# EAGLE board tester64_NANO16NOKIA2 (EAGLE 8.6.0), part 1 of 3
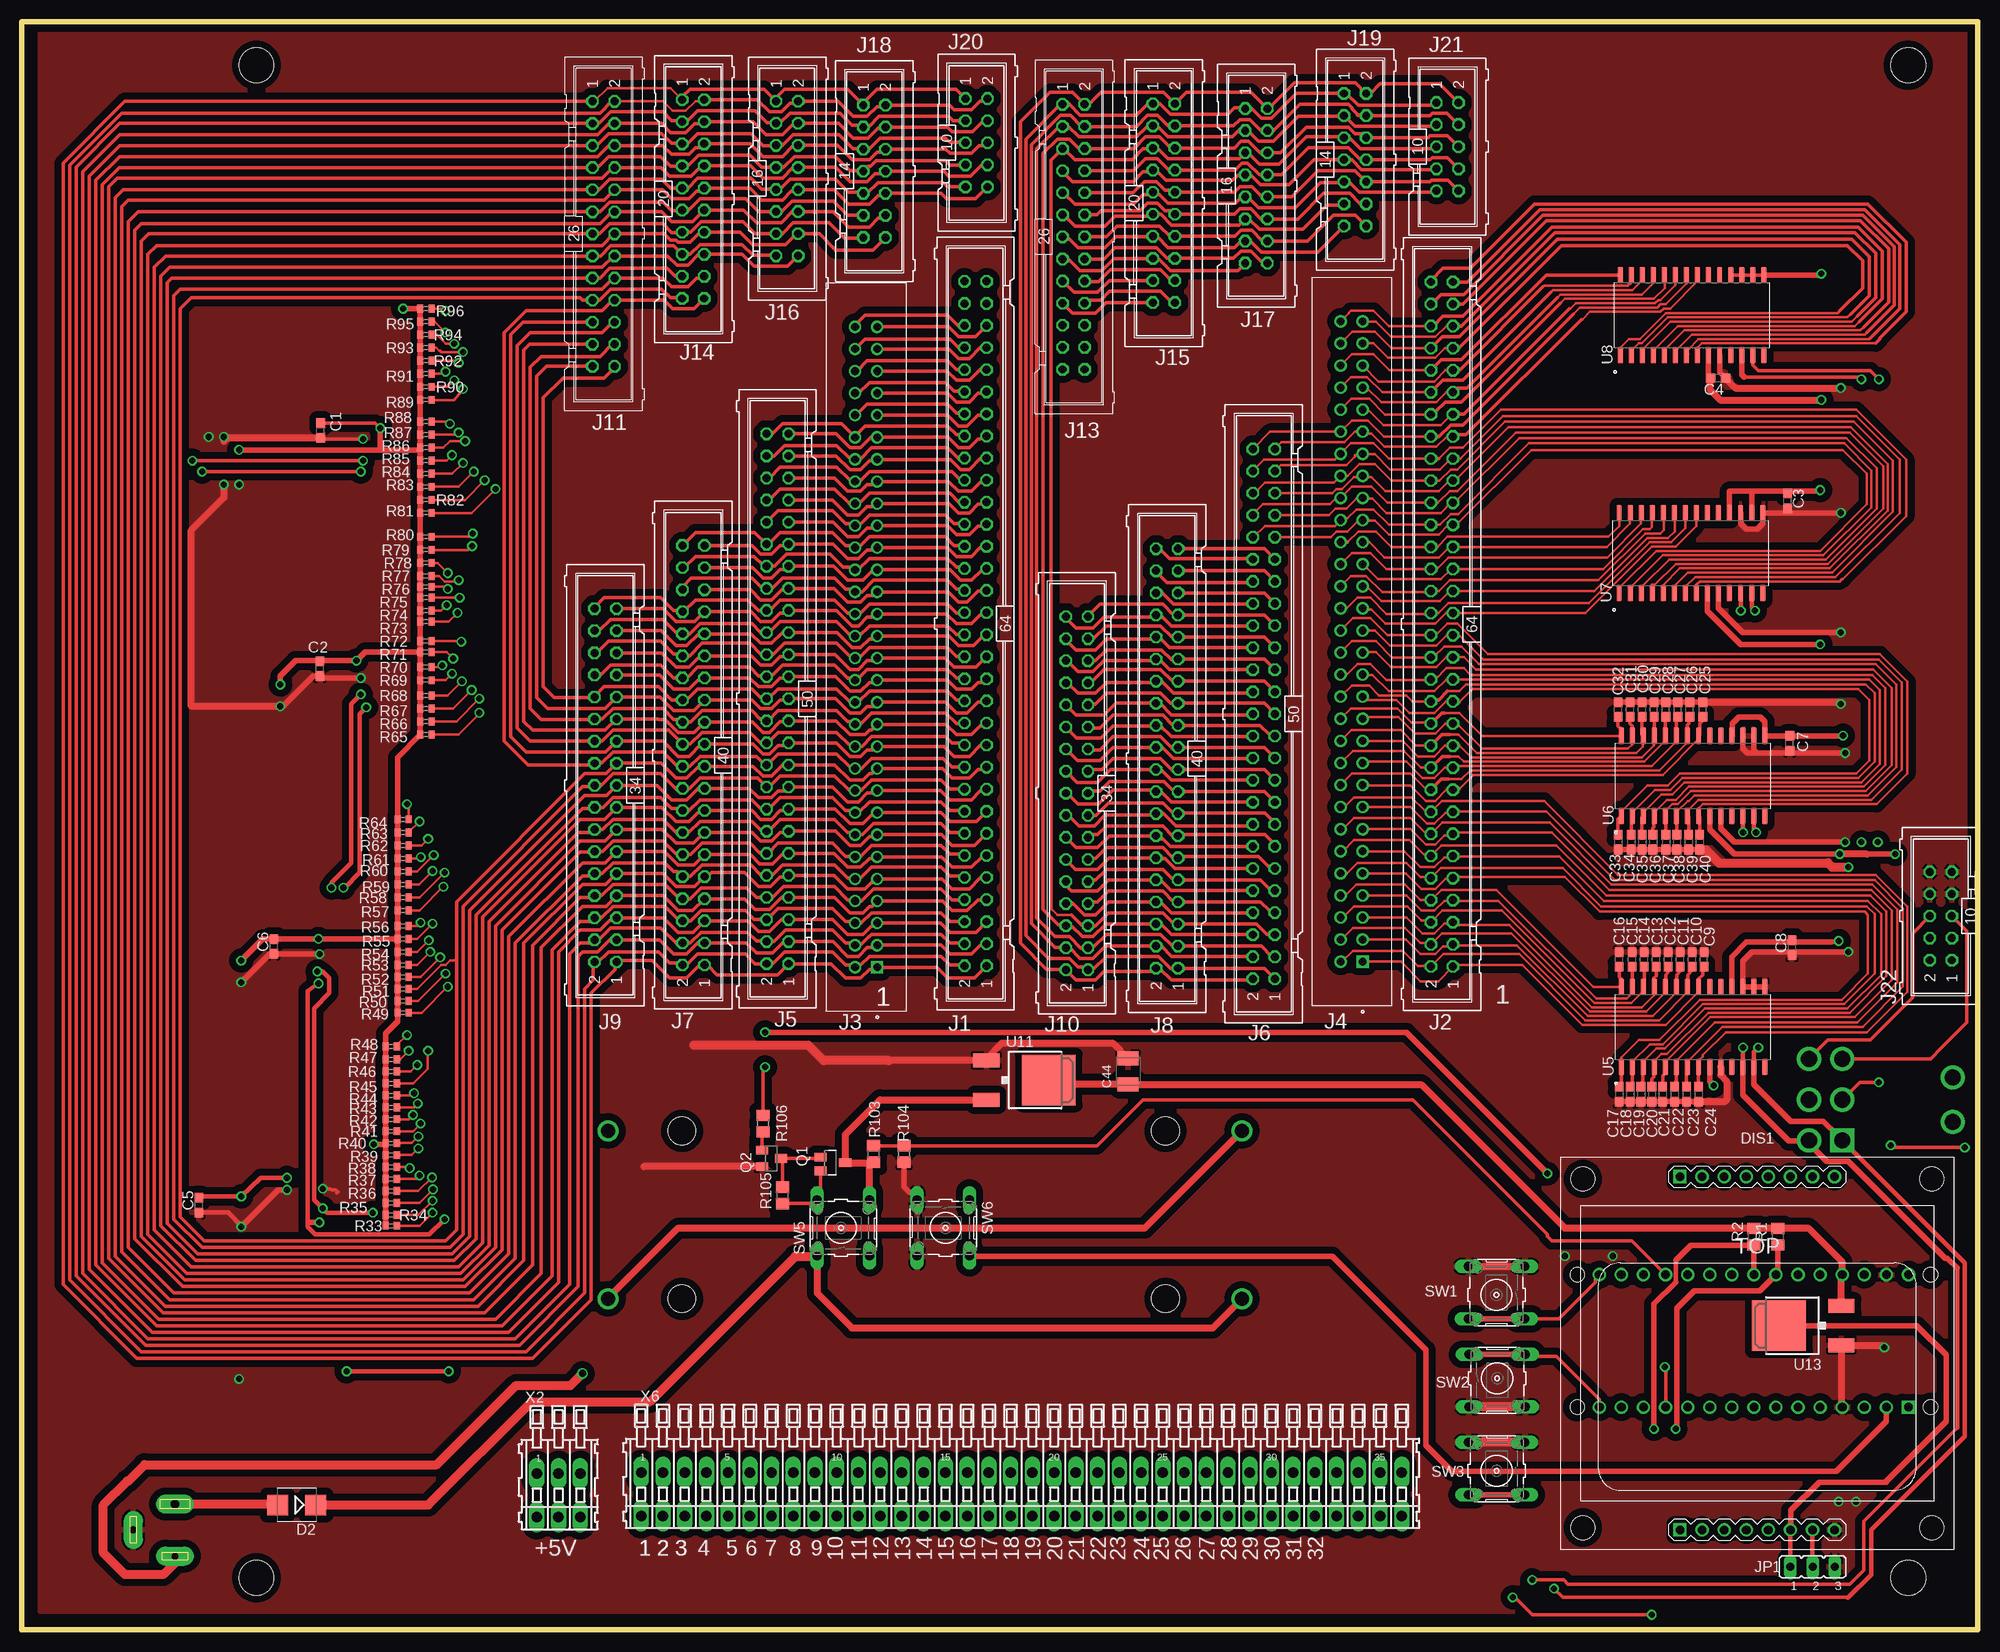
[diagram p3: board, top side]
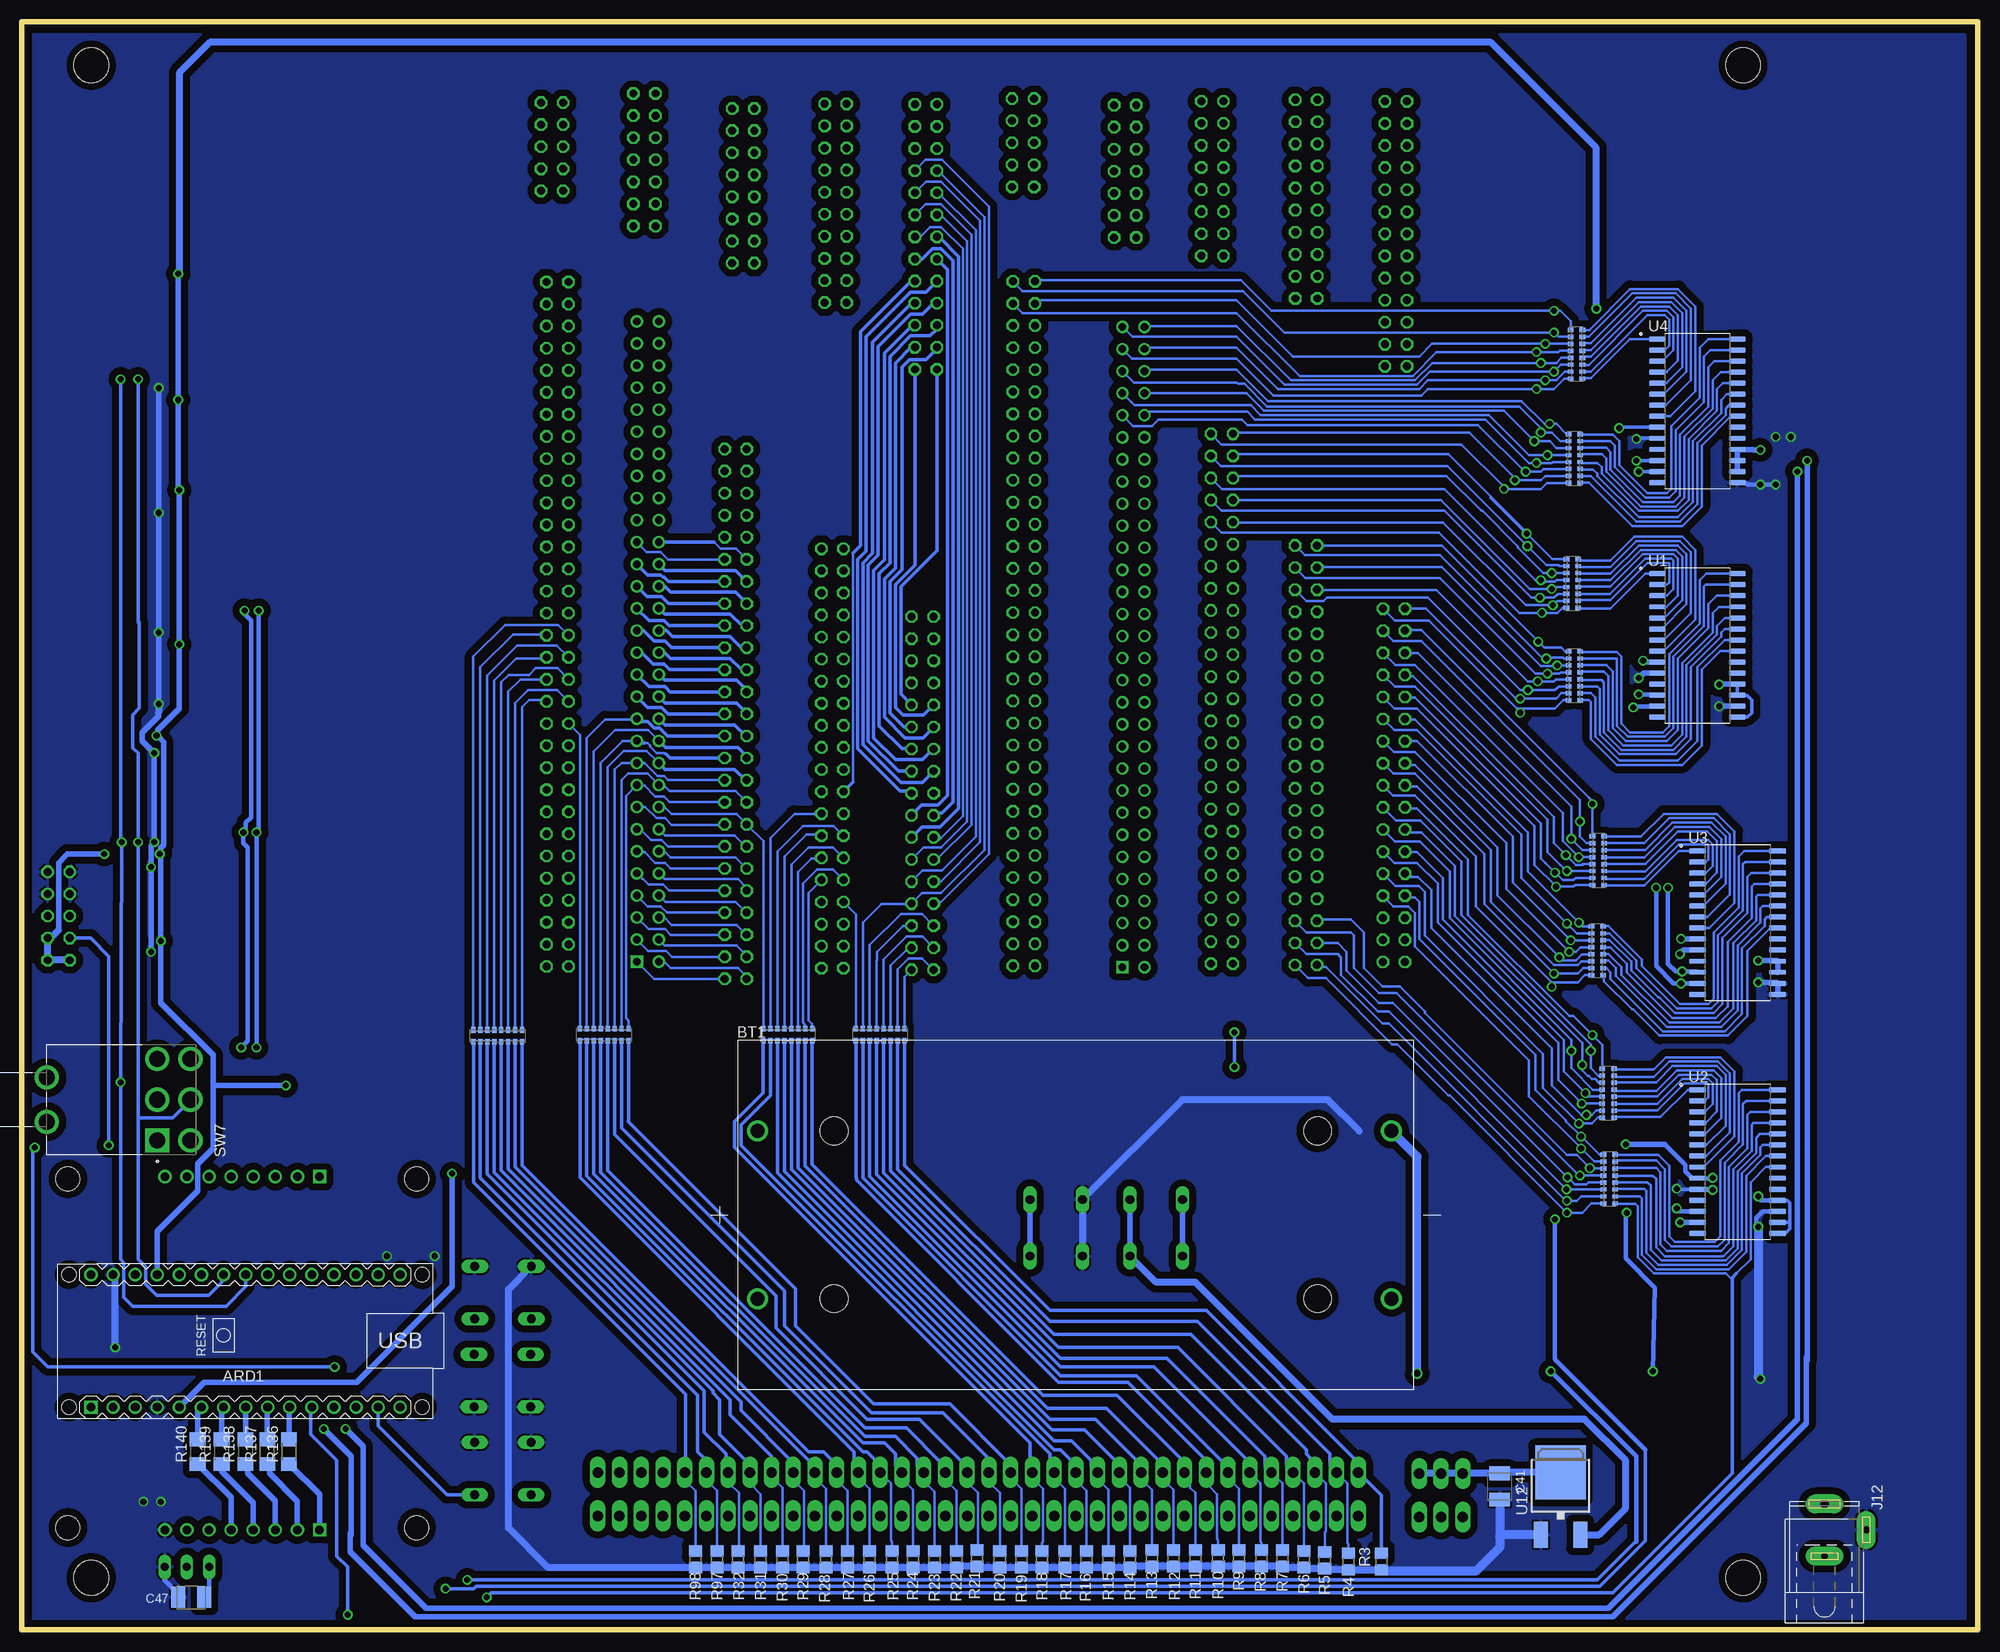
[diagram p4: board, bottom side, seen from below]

Size 225 x 185 mm. Coordinates in mm from the lower left corner, seen from the top.
Outline: 0,185 225,185 225,0 0,0 0,185
Copper layers (1*16): Top 0.035mm / dielectric 1.5mm / Bottom 0.035mm
Design rules "default *": minimum track width 10mil, minimum drill 24mil, track to track 5mil, track to pad 5mil, pad to pad 5mil, via to via 5mil, smd to smd 5mil, copper to edge 20mil, drill to drill 8mil, minimum pad ring 10mil, minimum via ring 8mil, stop-mask expansion 4mil, vias tented up to drill 0mil, thermal gap 10mil
Holes 4 mm at 27,6 217,6 27,180 217,180

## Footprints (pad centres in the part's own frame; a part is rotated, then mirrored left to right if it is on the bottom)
ARDUINO-NANO-3.0 = drill 1 square: J1.1 17.78,7.62 | drill 1: J1.2 15.24,7.62; J1.3 12.7,7.62; J1.4 10.16,7.62; J1.5 7.62,7.62; J1.6 5.08,7.62; J1.7 2.54,7.62; J1.8 0,7.62; J1.9 -2.54,7.62; J1.10 -5.08,7.62; J1.11 -7.62,7.62; J1.12 -10.16,7.62; J1.13 -12.7,7.62; J1.14 -15.24,7.62; J1.15 -17.78,7.62; J2.1 17.78,-7.62; J2.2 15.24,-7.62; J2.3 12.7,-7.62; J2.4 10.16,-7.62; J2.5 7.62,-7.62; J2.6 5.08,-7.62; J2.7 2.54,-7.62; J2.8 0,-7.62; J2.9 -2.54,-7.62; J2.10 -5.08,-7.62; J2.11 -7.62,-7.62; J2.12 -10.16,-7.62; J2.13 -12.7,-7.62; J2.14 -15.24,-7.62; J2.15 -17.78,-7.62 | hole 1.651: -20.32,7.62; -20.32,-7.62; 20.32,-7.62; 20.32,7.62
BAT_BK-18650-PC4 = drill 1.6: 1+ -36.6,9.65; 1- 36.3,9.65; 2+ -36.6,-9.65; 2- 36.3,-9.65 | hole 3.2: -27.81,-9.65; -27.81,9.65; 27.81,-9.65; 27.81,9.65
C0603 = smd 1.1 x 1: 1 -0.85,0; 2 0.85,0
SMC_B = smd 1.6 x 2.4: + -1.5,0; - 1.5,0
SMB = smd 2.4 x 2.4: A 2.2,0; C -2.2,0
DISPLAY-NOKIA-5110 = drill 1 square: J1.1 0,0; J2.1 0,40.64 | drill 1: J1.2 2.54,0; J1.3 5.08,0; J1.4 7.62,0; J1.5 10.16,0; J1.6 12.7,0; J1.7 15.24,0; J1.8 17.78,0; J2.2 2.54,40.64; J2.3 5.08,40.64; J2.4 7.62,40.64; J2.5 10.16,40.64; J2.6 12.7,40.64; J2.7 15.24,40.64; J2.8 17.78,40.64 | hole 2.8: -11.176,0.254; 28.956,0.254; 28.956,40.386; -11.176,40.386
ML64 = drill 0.914 octagon: 1 -39.37,-1.27; 2 -39.37,1.27; 3 -36.83,-1.27; 4 -36.83,1.27; 5 -34.29,-1.27; 6 -34.29,1.27; 7 -31.75,-1.27; 8 -31.75,1.27; 9 -29.21,-1.27; 10 -29.21,1.27; 11 -26.67,-1.27; 12 -26.67,1.27; 13 -24.13,-1.27; 14 -24.13,1.27; 15 -21.59,-1.27; 16 -21.59,1.27; 17 -19.05,-1.27; 18 -19.05,1.27; 19 -16.51,-1.27; 20 -16.51,1.27; 21 -13.97,-1.27; 22 -13.97,1.27; 23 -11.43,-1.27; 24 -11.43,1.27; 25 -8.89,-1.27; 26 -8.89,1.27; 27 -6.35,-1.27; 28 -6.35,1.27; 29 -3.81,-1.27; 30 -3.81,1.27; 31 -1.27,-1.27; 32 -1.27,1.27; 33 1.27,-1.27; 34 1.27,1.27; 35 3.81,-1.27; 36 3.81,1.27; 37 6.35,-1.27; 38 6.35,1.27; 39 8.89,-1.27; 40 8.89,1.27; 41 11.43,-1.27; 42 11.43,1.27; 43 13.97,-1.27; 44 13.97,1.27; 45 16.51,-1.27; 46 16.51,1.27; 47 19.05,-1.27; 48 19.05,1.27; 49 21.59,-1.27; 50 21.59,1.27; 51 24.13,-1.27; 52 24.13,1.27; 53 26.67,-1.27; 54 26.67,1.27; 55 29.21,-1.27; 56 29.21,1.27; 57 31.75,-1.27; 58 31.75,1.27; 59 34.29,-1.27; 60 34.29,1.27; 61 36.83,-1.27; 62 36.83,1.27; 63 39.37,-1.27; 64 39.37,1.27
TE_3-1761608-6 = drill 0.89 pad 1.24 square: 1 0,0 | drill 0.89 pad 1.24: 2 0,2.54; 3 2.54,0; 4 2.54,2.54; 5 5.08,0; 6 5.08,2.54; 7 7.62,0; 8 7.62,2.54; 9 10.16,0; 10 10.16,2.54; 11 12.7,0; 12 12.7,2.54; 13 15.24,0; 14 15.24,2.54; 15 17.78,0; 16 17.78,2.54; 17 20.32,0; 18 20.32,2.54; 19 22.86,0; 20 22.86,2.54; 21 25.4,0; 22 25.4,2.54; 23 27.94,0; 24 27.94,2.54; 25 30.48,0; 26 30.48,2.54; 27 33.02,0; 28 33.02,2.54; 29 35.56,0; 30 35.56,2.54; 31 38.1,0; 32 38.1,2.54; 33 40.64,0; 34 40.64,2.54; 35 43.18,0; 36 43.18,2.54; 37 45.72,0; 38 45.72,2.54; 39 48.26,0; 40 48.26,2.54; 41 50.8,0; 42 50.8,2.54; 43 53.34,0; 44 53.34,2.54; 45 55.88,0; 46 55.88,2.54; 47 58.42,0; 48 58.42,2.54; 49 60.96,0; 50 60.96,2.54; 51 63.5,0; 52 63.5,2.54; 53 66.04,0; 54 66.04,2.54; 55 68.58,0; 56 68.58,2.54; 57 71.12,0; 58 71.12,2.54; 59 73.66,0; 60 73.66,2.54
ML50 = drill 0.914 octagon: 1 -30.48,-1.27; 2 -30.48,1.27; 3 -27.94,-1.27; 4 -27.94,1.27; 5 -25.4,-1.27; 6 -25.4,1.27; 7 -22.86,-1.27; 8 -22.86,1.27; 9 -20.32,-1.27; 10 -20.32,1.27; 11 -17.78,-1.27; 12 -17.78,1.27; 13 -15.24,-1.27; 14 -15.24,1.27; 15 -12.7,-1.27; 16 -12.7,1.27; 17 -10.16,-1.27; 18 -10.16,1.27; 19 -7.62,-1.27; 20 -7.62,1.27; 21 -5.08,-1.27; 22 -5.08,1.27; 23 -2.54,-1.27; 24 -2.54,1.27; 25 0,-1.27; 26 0,1.27; 27 2.54,-1.27; 28 2.54,1.27; 29 5.08,-1.27; 30 5.08,1.27; 31 7.62,-1.27; 32 7.62,1.27; 33 10.16,-1.27; 34 10.16,1.27; 35 12.7,-1.27; 36 12.7,1.27; 37 15.24,-1.27; 38 15.24,1.27; 39 17.78,-1.27; 40 17.78,1.27; 41 20.32,-1.27; 42 20.32,1.27; 43 22.86,-1.27; 44 22.86,1.27; 45 25.4,-1.27; 46 25.4,1.27; 47 27.94,-1.27; 48 27.94,1.27; 49 30.48,-1.27; 50 30.48,1.27
ML40 = drill 0.914 octagon: 1 -24.13,-1.27; 2 -24.13,1.27; 3 -21.59,-1.27; 4 -21.59,1.27; 5 -19.05,-1.27; 6 -19.05,1.27; 7 -16.51,-1.27; 8 -16.51,1.27; 9 -13.97,-1.27; 10 -13.97,1.27; 11 -11.43,-1.27; 12 -11.43,1.27; 13 -8.89,-1.27; 14 -8.89,1.27; 15 -6.35,-1.27; 16 -6.35,1.27; 17 -3.81,-1.27; 18 -3.81,1.27; 19 -1.27,-1.27; 20 -1.27,1.27; 21 1.27,-1.27; 22 1.27,1.27; 23 3.81,-1.27; 24 3.81,1.27; 25 6.35,-1.27; 26 6.35,1.27; 27 8.89,-1.27; 28 8.89,1.27; 29 11.43,-1.27; 30 11.43,1.27; 31 13.97,-1.27; 32 13.97,1.27; 33 16.51,-1.27; 34 16.51,1.27; 35 19.05,-1.27; 36 19.05,1.27; 37 21.59,-1.27; 38 21.59,1.27; 39 24.13,-1.27; 40 24.13,1.27
ML34 = drill 0.914 octagon: 1 -20.32,-1.27; 2 -20.32,1.27; 3 -17.78,-1.27; 4 -17.78,1.27; 5 -15.24,-1.27; 6 -15.24,1.27; 7 -12.7,-1.27; 8 -12.7,1.27; 9 -10.16,-1.27; 10 -10.16,1.27; 11 -7.62,-1.27; 12 -7.62,1.27; 13 -5.08,-1.27; 14 -5.08,1.27; 15 -2.54,-1.27; 16 -2.54,1.27; 17 0,-1.27; 18 0,1.27; 19 2.54,-1.27; 20 2.54,1.27; 21 5.08,-1.27; 22 5.08,1.27; 23 7.62,-1.27; 24 7.62,1.27; 25 10.16,-1.27; 26 10.16,1.27; 27 12.7,-1.27; 28 12.7,1.27; 29 15.24,-1.27; 30 15.24,1.27; 31 17.78,-1.27; 32 17.78,1.27; 33 20.32,-1.27; 34 20.32,1.27
ML26 = drill 0.914 octagon: 1 -15.24,-1.27; 2 -15.24,1.27; 3 -12.7,-1.27; 4 -12.7,1.27; 5 -10.16,-1.27; 6 -10.16,1.27; 7 -7.62,-1.27; 8 -7.62,1.27; 9 -5.08,-1.27; 10 -5.08,1.27; 11 -2.54,-1.27; 12 -2.54,1.27; 13 0,-1.27; 14 0,1.27; 15 2.54,-1.27; 16 2.54,1.27; 17 5.08,-1.27; 18 5.08,1.27; 19 7.62,-1.27; 20 7.62,1.27; 21 10.16,-1.27; 22 10.16,1.27; 23 12.7,-1.27; 24 12.7,1.27; 25 15.24,-1.27; 26 15.24,1.27
SPC4078 = drill 0.8 pad 2.184 long: 1 -3,0; 2 0,-4.8 | drill 1 pad 2.184 long: 3 3,0
ML20 = drill 0.914 octagon: 1 -11.43,-1.27; 2 -11.43,1.27; 3 -8.89,-1.27; 4 -8.89,1.27; 5 -6.35,-1.27; 6 -6.35,1.27; 7 -3.81,-1.27; 8 -3.81,1.27; 9 -1.27,-1.27; 10 -1.27,1.27; 11 1.27,-1.27; 12 1.27,1.27; 13 3.81,-1.27; 14 3.81,1.27; 15 6.35,-1.27; 16 6.35,1.27; 17 8.89,-1.27; 18 8.89,1.27; 19 11.43,-1.27; 20 11.43,1.27
ML16 = drill 0.914 octagon: 1 -8.89,-1.27; 2 -8.89,1.27; 3 -6.35,-1.27; 4 -6.35,1.27; 5 -3.81,-1.27; 6 -3.81,1.27; 7 -1.27,-1.27; 8 -1.27,1.27; 9 1.27,-1.27; 10 1.27,1.27; 11 3.81,-1.27; 12 3.81,1.27; 13 6.35,-1.27; 14 6.35,1.27; 15 8.89,-1.27; 16 8.89,1.27
ML14 = drill 0.914 octagon: 1 -7.62,-1.27; 2 -7.62,1.27; 3 -5.08,-1.27; 4 -5.08,1.27; 5 -2.54,-1.27; 6 -2.54,1.27; 7 0,-1.27; 8 0,1.27; 9 2.54,-1.27; 10 2.54,1.27; 11 5.08,-1.27; 12 5.08,1.27; 13 7.62,-1.27; 14 7.62,1.27
ML10 = drill 0.914 octagon: 1 -5.08,-1.27; 2 -5.08,1.27; 3 -2.54,-1.27; 4 -2.54,1.27; 5 0,-1.27; 6 0,1.27; 7 2.54,-1.27; 8 2.54,1.27; 9 5.08,-1.27; 10 5.08,1.27
JP2 = drill 0.914 long: 1 -2.54,0; 2 0,0; 3 2.54,0
SOT23 = smd 1 x 1.4: 1 0,1.735; 2 -0.632,-1.1; 3 0.95,-1.1
SOT23' = smd 1 x 1.4: 1 -0.95,-1.1; 2 0.95,-1.1; 3 0,1.1
R0805 = smd 1.3 x 1.5: 1 -0.95,0; 2 0.95,0
R0402 = smd 0.7 x 0.9: 1 -0.65,0; 2 0.65,0
R1206 = smd 1.6 x 1.803: 1 -1.422,0; 2 1.422,0
CAY16Y8 = smd 0.5 x 0.65: 1 -3.8,0.225; 2 -3,0.225; 3 -2.2,0.225; 4 -1.4,0.225; 5 -0.6,0.225; 6 0.2,0.225; 7 1,0.225; 8 1.8,0.225; 9 -3.8,1.575; 10 -3,1.575; 11 -2.2,1.575; 12 -1.4,1.575; 13 -0.6,1.575; 14 0.2,1.575; 15 1,1.575; 16 1.8,1.575
B3F-10XX = drill 1.016 long: 1 -3.251,2.761; 2 3.251,2.761; 3 -3.251,-3.261; 4 3.251,-3.261
SW_100DP1T2B4M6QE = drill 1.85 square: 1 -4.7,1.905 | drill 1.85: 2 0,1.905; 3 4.7,1.905; 4 -4.7,-1.905; 5 0,-1.905; 6 4.7,-1.905; S1 -2.54,14.605; S2 2.54,14.605
SOIC127P1030X265-28N = smd 1.9 x 0.6: 1 -4.605,8.255; 2 -4.605,6.985; 3 -4.605,5.715; 4 -4.605,4.445; 5 -4.605,3.175; 6 -4.605,1.905; 7 -4.605,0.635; 8 -4.605,-0.635; 9 -4.605,-1.905; 10 -4.605,-3.175; 11 -4.605,-4.445; 12 -4.605,-5.715; 13 -4.605,-6.985; 14 -4.605,-8.255; 15 4.605,-8.255; 16 4.605,-6.985; 17 4.605,-5.715; 18 4.605,-4.445; 19 4.605,-3.175; 20 4.605,-1.905; 21 4.605,-0.635; 22 4.605,0.635; 23 4.605,1.905; 24 4.605,3.175; 25 4.605,4.445; 26 4.605,5.715; 27 4.605,6.985; 28 4.605,8.255
DPACK = smd 1.6 x 3: 1 -2.28,-4.8; 3 2.28,-4.8 | smd 5.8 x 6.2: 4 0,2.38
234-203 = drill 1.2 long: A1 -2.5,2.5; A2 0,2.5; A3 2.5,2.5; B1 -2.5,-2.5; B2 0,-2.5; B3 2.5,-2.5
234-236 = drill 1.2 long: A1 -43.75,2.5; A2 -41.25,2.5; A3 -38.75,2.5; A4 -36.25,2.5; A5 -33.75,2.5; A6 -31.25,2.5; A7 -28.75,2.5; A8 -26.25,2.5; A9 -23.75,2.5; A10 -21.25,2.5; A11 -18.75,2.5; A12 -16.25,2.5; A13 -13.75,2.5; A14 -11.25,2.5; A15 -8.75,2.5; A16 -6.25,2.5; A17 -3.75,2.5; A18 -1.25,2.5; A19 1.25,2.5; A20 3.75,2.5; A21 6.25,2.5; A22 8.75,2.5; A23 11.25,2.5; A24 13.75,2.5; A25 16.25,2.5; A26 18.75,2.5; A27 21.25,2.5; A28 23.75,2.5; A29 26.25,2.5; A30 28.75,2.5; A31 31.25,2.5; A32 33.75,2.5; A33 36.25,2.5; A34 38.75,2.5; A35 41.25,2.5; A36 43.75,2.5; B1 -43.75,-2.5; B2 -41.25,-2.5; B3 -38.75,-2.5; B4 -36.25,-2.5; B5 -33.75,-2.5; B6 -31.25,-2.5; B7 -28.75,-2.5; B8 -26.25,-2.5; B9 -23.75,-2.5; B10 -21.25,-2.5; B11 -18.75,-2.5; B12 -16.25,-2.5; B13 -13.75,-2.5; B14 -11.25,-2.5; B15 -8.75,-2.5; B16 -6.25,-2.5; B17 -3.75,-2.5; B18 -1.25,-2.5; B19 1.25,-2.5; B20 3.75,-2.5; B21 6.25,-2.5; B22 8.75,-2.5; B23 11.25,-2.5; B24 13.75,-2.5; B25 16.25,-2.5; B26 18.75,-2.5; B27 21.25,-2.5; B28 23.75,-2.5; B29 26.25,-2.5; B30 28.75,-2.5; B31 31.25,-2.5; B32 33.75,-2.5; B33 36.25,-2.5; B34 38.75,-2.5; B35 41.25,-2.5; B36 43.75,-2.5

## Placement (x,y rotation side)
ARD1  ARDUINO-NANO-3.0  [ARDUINO-NANO-3.0]  199.25,33.25 180 bottom
BT1  BK-18650-PC4  [BAT_BK-18650-PC4]  103.75,47.75 0 bottom
C1  [C0603]  34.38,137.98 90 top
C2  [C0603]  34.31,110.58 90 top
C3  [C0603]  203.12,129.88 90 top
C4  [C0603]  195.12,144 180 top
C5  [C0603]  20.38,48.88 90 top
C6  [C0603]  29,78.62 90 top
C7  [C0603]  203.38,102 90 top
C8  [C0603]  203.62,78.5 90 top
C9  [C0603]  193.5,77.12 90 top
C10  [C0603]  192.12,77.12 90 top
C11  [C0603]  190.75,77.12 90 top
C12  [C0603]  189.38,77.12 90 top
C13  [C0603]  188,77.12 90 top
C14  [C0603]  186.62,77.12 90 top
C15  [C0603]  185.25,77.12 90 top
C16  [C0603]  183.75,77.12 90 top
C17  [C0603]  183.75,61.62 270 top
C18  [C0603]  185,61.62 270 top
C19  [C0603]  186.25,61.62 270 top
C20  [C0603]  187.5,61.62 270 top
C21  [C0603]  188.75,61.62 270 top
C22  [C0603]  190.12,61.62 270 top
C23  [C0603]  191.5,61.62 270 top
C24  [C0603]  192.88,61.62 270 top
C25  [C0603]  193.38,105.88 90 top
C26  [C0603]  191.88,105.88 90 top
C27  [C0603]  190.5,105.88 90 top
C28  [C0603]  189.12,105.88 90 top
C29  [C0603]  187.75,105.88 90 top
C30  [C0603]  186.38,105.88 90 top
C31  [C0603]  185,105.88 90 top
C32  [C0603]  183.62,105.88 90 top
C33  [C0603]  183.62,90.62 270 top
C34  [C0603]  185.12,90.62 270 top
C35  [C0603]  186.38,90.62 270 top
C36  [C0603]  187.62,90.62 270 top
C37  [C0603]  189.12,90.62 270 top
C38  [C0603]  190.38,90.62 270 top
C39  [C0603]  191.75,90.62 270 top
C40  [C0603]  193,90.62 270 top
C41  [SMC_B]  55,16.5 270 bottom
C44  [SMC_B]  127.25,64.25 90 top
C47  [SMC_B]  205.5,3.75 180 bottom
D2  [SMB]  31.62,14.38 180 top
DIS1  DISPLAY-NOKIA-5110  [DISPLAY-NOKIA-5110]  190.75,11.5 0 top
J1  [ML64]  109.72,115.76 90 top
J2  [ML64]  163.38,115.7 90 top
J3  3-1761608-6  [TE_3-1761608-6]  98.4,76.24 90 top
J4  3-1761608-6  [TE_3-1761608-6]  154.25,76.88 90 top
J5  [ML50]  86.94,107.12 90 top
J6  [ML50]  142.88,105.38 90 top
J7  [ML40]  77.26,100.62 90 top
J8  [ML40]  131.75,100.25 90 top
J9  [ML34]  67.14,97.16 90 top
J10  [ML34]  121.38,96.25 90 top
J11  [ML26]  66.92,160.6 270 top
J12  [SPC4078]  17.62,11.5 90 bottom
J13  [ML26]  121,160.25 270 top
J14  [ML20]  77.24,164.6 270 top
J15  [ML20]  131.38,164.12 270 top
J16  [ML16]  88.05,166.97 270 top
J17  [ML16]  142,166.12 270 top
J18  [ML14]  98.07,167.8 270 top
J19  [ML14]  153.38,169.12 270 top
J20  [ML10]  109.82,171.08 270 top
J21  [ML10]  164,170.62 270 top
J22  [ML10]  220.75,82.12 90 top
JP1  [JP2]  206,7.25 0 top
Q1  STR2P3LLH6  [SOT23]  93,53.75 270 top
Q2  BC846  [SOT23']  86.25,54.25 270 top
R1  [R0805]  202,45.25 90 top
R2  [R0805]  199.25,45.25 90 top
R3  [R0805]  68.62,7.88 90 bottom
R4  [R0805]  72.38,7.88 90 bottom
R5  [R0805]  75.12,8 90 bottom
R6  [R0805]  77.5,8.12 90 bottom
R7  [R0805]  80,8.25 90 bottom
R8  [R0805]  82.38,8.25 90 bottom
R9  [R0805]  85,8.25 90 bottom
R10  [R0805]  87.38,8.25 90 bottom
R11  [R0805]  90,8.25 90 bottom
R12  [R0805]  92.5,8.25 90 bottom
R13  [R0805]  95,8.25 90 bottom
R14  [R0805]  97.5,8.12 90 bottom
R15  [R0805]  100,8.12 90 bottom
R16  [R0805]  102.5,8.12 90 bottom
R17  [R0805]  105,8.12 90 bottom
R18  [R0805]  107.62,8.12 90 bottom
R19  [R0805]  110,8.12 90 bottom
R20  [R0805]  112.5,8.12 90 bottom
R21  [R0805]  115.12,8.25 90 bottom
R22  [R0805]  117.5,8.12 90 bottom
R23  [R0805]  120,8.12 90 bottom
R24  [R0805]  122.5,8.12 90 bottom
R25  [R0805]  124.88,8.12 90 bottom
R26  [R0805]  127.5,8.12 90 bottom
R27  [R0805]  130,8.12 90 bottom
R28  [R0805]  132.5,8.12 90 bottom
R29  [R0805]  135.12,8.12 90 bottom
R30  [R0805]  137.5,8.12 90 bottom
R31  [R0805]  140,8.12 90 bottom
R32  [R0805]  142.62,8.12 90 bottom
R33  [R0402]  42.5,46.5 180 top
R34  [R0402]  42.5,47.75 180 top
R35  [R0402]  42.5,49.12 180 top
R36  [R0402]  42.5,50.5 180 top
R37  [R0402]  42.5,51.88 180 top
R38  [R0402]  42.5,53.25 180 top
R39  [R0402]  42.5,54.62 180 top
R40  [R0402]  42.5,56 180 top
R41  [R0402]  42.5,57.38 180 top
R42  [R0402]  42.5,58.75 180 top
R43  [R0402]  42.5,60.12 180 top
R44  [R0402]  42.5,61.5 180 top
R45  [R0402]  42.5,62.88 180 top
R46  [R0402]  42.5,64.25 180 top
R47  [R0402]  42.5,65.62 180 top
R48  [R0402]  42.5,67.12 180 top
R49  [R0402]  43.88,71 180 top
R50  [R0402]  43.88,72.38 180 top
R51  [R0402]  43.88,73.75 180 top
R52  [R0402]  43.88,75.12 180 top
R53  [R0402]  43.88,76.5 180 top
R54  [R0402]  43.88,78 180 top
R55  [R0402]  43.88,79.5 180 top
R56  [R0402]  43.88,81 180 top
R57  [R0402]  43.88,82.75 180 top
R58  [R0402]  43.88,84.25 180 top
R59  [R0402]  43.88,85.75 180 top
R60  [R0402]  43.88,87.25 180 top
R61  [R0402]  43.88,88.75 180 top
R62  [R0402]  43.88,90.25 180 top
R63  [R0402]  43.88,91.75 180 top
R64  [R0402]  43.88,93.25 180 top
R65  [R0402]  46.5,103 180 top
R66  [R0402]  46.5,104.5 180 top
R67  [R0402]  46.5,106 180 top
R68  [R0402]  46.5,107.5 180 top
R69  [R0402]  46.5,109.25 180 top
R70  [R0402]  46.5,110.75 180 top
R71  [R0402]  46.5,112.5 180 top
R72  [R0402]  46.5,113.75 180 top
R73  [R0402]  46.5,116 180 top
R74  [R0402]  46.5,117.25 180 top
R75  [R0402]  46.5,118.75 180 top
R76  [R0402]  46.5,120 180 top
R77  [R0402]  46.5,121.25 180 top
R78  [R0402]  46.5,122.75 180 top
R79  [R0402]  46.5,124.25 180 top
R80  [R0402]  46.5,125.75 180 top
R81  [R0402]  46.5,128.5 180 top
R82  [R0402]  46.5,130 180 top
R83  [R0402]  46.5,131.5 180 top
R84  [R0402]  46.5,133 180 top
R85  [R0402]  46.5,134.5 180 top
R86  [R0402]  46.5,136 180 top
R87  [R0402]  46.5,137.5 180 top
R88  [R0402]  46.5,139 180 top
R89  [R0402]  46.5,141.5 180 top
R90  [R0402]  46.5,143 180 top
R91  [R0402]  46.5,144.5 180 top
R92  [R0402]  46.5,146 180 top
R93  [R0402]  46.5,147.5 180 top
R94  [R0402]  46.5,149 180 top
R95  [R0402]  46.5,150.5 180 top
R96  [R0402]  46.5,152 180 top
R97  [R0805]  145,8.12 90 bottom
R98  [R0805]  147.5,8.12 90 bottom
R103  [R0805]  98,54.75 90 top
R104  [R0805]  101.5,54.75 270 top
R105  [R0805]  87.5,50 90 top
R106  [R0805]  85.25,58.25 270 top
R136  [R1206]  194.25,20.5 90 bottom
R137  [R1206]  196.75,20.5 90 bottom
R138  [R1206]  199.25,20.5 90 bottom
R139  [R1206]  202,20.5 90 bottom
R140  [R1206]  204.75,20.5 90 bottom
RN1  CAY16-J8  [CAY16Y8]  41.5,52.88 90 bottom
RN2  CAY16-J8  [CAY16Y8]  41.62,62.75 90 bottom
RN3  CAY16-J8  [CAY16Y8]  42.88,79.12 90 bottom
RN4  CAY16-J8  [CAY16Y8]  42.75,89.5 90 bottom
RN5  CAY16-J8  [CAY16Y8]  45.5,110.75 90 bottom
RN6  CAY16-J8  [CAY16Y8]  45.75,121.38 90 bottom
RN7  CAY16-J8  [CAY16Y8]  45.5,135.75 90 bottom
RN8  CAY16-J8  [CAY16Y8]  45.25,147.75 90 bottom
RN9  CAY16-J8  [CAY16Y8]  127.25,69.38 180 bottom
RN10  CAY16-J8  [CAY16Y8]  137.88,69.38 180 bottom
RN11  CAY16-J8  [CAY16Y8]  159,69.38 180 bottom
RN12  CAY16-J8  [CAY16Y8]  171.25,69.25 180 bottom
SW1  [B3F-10XX]  169.64,38.56 180 top
SW2  [B3F-10XX]  169.73,28.94 0 top
SW3  [B3F-10XX]  169.66,18.31 180 top
SW5  [B3F-10XX]  94.25,46.25 90 top
SW6  [B3F-10XX]  106.25,46.25 270 top
SW7  100DP1T2B4M6QE  [SW_100DP1T2B4M6QE]  207.5,61 90 bottom
U1  MCP23017-E/SO  [SOIC127P1030X265-28N]  32.25,113.25 0 bottom
U2  MCP23017-E/SO  [SOIC127P1030X265-28N]  27.62,53.88 0 bottom
U3  MCP23017-E/SO  [SOIC127P1030X265-28N]  27.62,81.38 0 bottom
U4  MCP23017-E/SO  [SOIC127P1030X265-28N]  32.25,140.25 0 bottom
U5  MCP23017-E/SO  [SOIC127P1030X265-28N]  192.25,69.38 90 top
U6  MCP23017-E/SO  [SOIC127P1030X265-28N]  192.25,98.25 90 top
U7  MCP23017-E/SO  [SOIC127P1030X265-28N]  192,123.88 90 top
U8  MCP23017-E/SO  [SOIC127P1030X265-28N]  192.12,151.25 90 top
U11  LD117ADT12TR  [DPACK]  115.75,63.25 270 top
U12  LD117ADT12TR  [DPACK]  48,15.75 0 bottom
U13  LD117ADT12TR  [DPACK]  204.5,35 90 top
X2  [234-203]  61.75,15.5 0 top
X6  [234-236]  115,15.62 0 top

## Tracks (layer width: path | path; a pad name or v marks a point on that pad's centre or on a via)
01  (via drill 0.7)
  Top 0.305: R33.1 45.75,46.5 v47.25,48 | J11.1 65.84,175.84 67.38,177.38 74.63,177.38 J14.1
  Top 0.406: J11.1 11.84,175.84 4.75,168.75 4.75,39.75 13.25,31.25 58.75,31.25 65.5,38 65.5,73.25 68.25,76 68.25,76.68 J9.1 68.57,77 72.5,77 74.5,75 76.5,75 77.99,76.49 J7.1 78.89,76.49 80,75.38 86.95,75.38 J5.1 93.11,76.64 94.75,75 96.5,75 97.5,76 98.16,76 J3.1 105.26,76.24 106.5,75 109.6,75 J1.1 | J14.1 75.97,176.35 76.88,177.25 85.38,177.25 J16.1 86.78,176.28 87.75,177.25 94.97,177.25 J18.1 96.8,175.68 98.38,177.25 107.46,177.25 J20.1
  Bottom 0.305: J7.1 77.04,75 75,75 67.38,67.38 66.75,67.38 60.88,61.5 60.75,61.5 v47.25,48 45.5,48 44.42,49.08 RN1.9
02  (via drill 0.7)
  Top 0.305: R34.1 45.62,47.75 v47.25,49.38 | J11.2 73.79,175.84 74.88,174.75 76.38,174.75 77.5,175.88 78.35,175.88 J14.2
  Top 0.406: J11.2 67.84,175.84 66.5,174.5 11.5,174.5 5.5,168.5 5.5,40.25 13.75,32 58,32 64.75,38.75 64.75,73.75 65.75,74.75 65.75,76.72 J9.2 66,76.71 66.21,76.71 67.5,78 73.25,78 74.5,76.75 75.73,76.75 J7.2 76.49,76.49 77.75,77.75 83.25,77.75 84.38,76.62 85.66,76.62 J5.2 85.67,76.67 86.42,76.67 87.75,78 93.25,78 94.75,76.5 95.59,76.5 J3.2 96.12,76.5 96.5,76.5 97.5,77.5 105.75,77.5 106.75,76.5 108.34,76.5 J1.2 | J14.2 84.59,176.03 86,174.62 87.38,174.62 88.38,175.62 89.08,175.62 J16.2 93.89,175.86 95.62,174.12 97.25,174.12 98.38,175.25 99.17,175.25 J18.2 106.7,175.42 107.25,174.88 109.25,174.88 110.25,175.88 110.81,175.88 J20.2
  Bottom 0.305: RN1.10 45.62,49.88 46.12,49.38 v47.25,49.38 47.38,49.38 67.75,69.75 68.5,69.75 75,76.25 75.75,76.25 J7.2
03  (via drill 0.7)
  Top 0.305: R35.1 45.75,49.12 v47.3,50.67
  Top 0.406: J1.3 110.81,78.75 110.25,78.75 109.25,77.75 106.75,77.75 105.72,78.78 J3.3 98.12,78.5 97.25,78.5 96.25,77.5 95,77.5 93.32,79.18 J5.3 88.16,79.12 87.62,79.12 86.38,77.88 84.5,77.88 83.35,79.03 J7.3 78.5,79 77.75,79 76.5,77.75 75,77.75 73.37,79.38 J9.3 67.63,79.38 66.25,78 64.5,78 64,77.5 64,39.5 57.25,32.75 14.25,32.75 6.25,40.75 6.25,168.25 11.3,173.3 J11.3 66.42,173.3 67.75,174.62 73.75,174.62 74.75,173.62 75.84,173.62 J14.3 76.49,173.49 77.75,174.75 84.38,174.75 85.75,173.38 86.72,173.38 J16.3 87.19,173.32 88.38,174.5 94.12,174.5 95.5,173.12 96.56,173.12 J18.3 97.38,172.88 98.62,174.12 106.62,174.12 107.12,173.62 J20.3
  Bottom 0.305: RN1.11 v47.3,50.67 67.75,71.12 69,71.12 73.25,75.38 73.25,77.38 73.62,77.75 77.25,77.75 J7.3
04  (via drill 0.7)
  Top 0.305: R36.1 45.62,50.5 v47.19,52.06
  Top 0.406: J1.4 108.38,79 106.75,79 105.75,80 97.75,80 97.5,79.75 97.47,79.75 96.5,78.78 J3.4 95.63,79 94.75,79 93.25,80.5 87.88,80.5 86.55,79.18 J5.4 85.6,79.25 84.5,79.25 83.5,80.25 78.12,80.25 76.9,79.03 J7.4 75.96,79 75.25,79 73.5,80.75 67.75,80.75 66.38,79.38 J9.4 65.49,79 64.25,79 63,77.75 63,39.75 56.75,33.5 14.5,33.5 7,41 7,167.75 11.25,172 66.25,172 67.55,173.3 J11.4 73.58,173.3 74.62,172.25 76.38,172.25 77.38,173.25 78.27,173.25 J14.4 84.13,173.49 85.62,172 87.5,172 88.62,173.12 89.12,173.12 J16.4 93.93,173.32 95.62,171.62 97.38,171.62 98.5,172.75 99.21,172.75 J18.4 106.49,172.88 107,172.38 109.38,172.38 110.38,173.38 110.85,173.38 J20.4
  Bottom 0.305: RN1.12 44.77,51.48 45,51.25 46.38,51.25 v47.19,52.06 67.25,72.12 68.88,72.12 72.62,75.88 72.62,78 73.62,79 75.96,79 J7.4
05  (via drill 0.7)
  Top 0.305: R37.1 45.35,51.88 v45.75,52.27
  Top 0.406: J1.5 110.97,81.47 109.75,80.25 106.75,80.25 105.68,81.32 J3.5 98.08,81 97.75,81 96.75,80 95,80 93.28,81.72 J5.5 88.18,81.75 87.38,81.75 86,80.38 84.75,80.38 83.56,81.57 J7.5 77.21,80.25 75.5,80.25 73.83,81.92 J9.5 68.24,81.75 67.75,81.75 66.5,80.5 64.25,80.5 61.75,78 61.75,40 56,34.25 15,34.25 7.75,41.5 7.75,167.25 11.26,170.76 J11.5 66.13,170.76 67.5,172.12 73.62,172.12 74.75,171 75.92,171 J14.5 76.58,170.95 77.75,172.12 83.88,172.12 85.25,170.75 86.75,170.75 J16.5 87.53,170.78 88.75,172 94,172 95.62,170.38 96.77,170.38 J18.5 97.47,170.34 98.75,171.62 106.25,171.62 106.75,171.12 108.5,171.12 J20.5
  Bottom 0.305: RN1.13 v45.75,52.27 45.9,52.27 66.88,73.25 68.88,73.25 71.75,76.12 71.75,79.88 72.12,80.25 77.21,80.25 J7.5
06  (via drill 0.7)
  Top 0.305: R38.1 44.5,53.25 v44.62,53.12
  Top 0.406: J1.6 108.42,81.5 106.75,81.5 105.75,82.5 97.75,82.5 96.57,81.32 J3.6 95.67,81.5 94.75,81.5 93.25,83 87,83 85.72,81.72 J5.6 85.64,81.75 84.25,81.75 83.25,82.75 78.12,82.75 76.94,81.57 J7.6 75.81,81.75 75.5,81.75 74,83.25 68,83.25 66.67,81.92 J9.6 65.45,81.5 64.25,81.5 61,78.25 61,40.75 55.25,35 15.5,35 8.5,42 8.5,166.75 11.25,169.5 66.25,169.5 67.51,170.76 J11.6 73.74,170.76 74.75,169.75 76.75,169.75 77.5,170.5 78.06,170.5 J14.6 83.8,170.95 85.25,169.5 87.5,169.5 88.78,170.78 J16.6 93.85,170.78 95.5,169.12 97.5,169.12 98.38,170 99,170 J18.6 106.28,170.34 106.75,169.88 109.25,169.88 110.12,170.75 110.77,170.75 J20.6
  Bottom 0.305: RN1.14 44.58,53.08 v44.62,53.12 46.12,54.62 47.25,54.62 63.62,71 63.62,71.12 66.5,74 68.5,74 70.62,76.12 70.62,80.25 72.12,81.75 75.81,81.75 J7.6
07  (via drill 0.7)
  Top 0.305: R39.1 44.88,54.62 v45.62,55.38
  Top 0.406: J1.7 110.98,84 110,84 108.75,82.75 107,82.75 105.89,83.86 J3.7 97.79,83.25 97.5,83.25 96.75,82.5 95.25,82.5 93.49,84.26 J5.7 87.38,84.25 86,82.88 84.38,82.88 83.14,84.11 J7.7 77.17,82.75 75.5,82.75 73.79,84.46 J9.7 67.2,83.25 64.5,83.25 59.75,78.5 59.75,41 54.5,35.75 15.75,35.75 9.25,42.25 9.25,166.25 11.22,168.22 J11.7 66.22,168.22 67.5,169.5 73.5,169.5 74.62,168.38 75.93,168.38 J14.7 76.66,168.41 77.88,169.62 83.75,169.62 85.12,168.25 86.76,168.25 J16.7 87.61,168.24 88.88,169.5 93.62,169.5 95.25,167.88 96.73,167.88 J18.7 97.38,168.38 97.62,168.38 98.25,169 106.25,169 106.75,168.5 108.52,168.5 J20.7
  Bottom 0.305: RN1.15 44.12,53.88 v45.62,55.38 51.62,61.38 51.62,65.5 64.75,78.62 64.75,82.5 65.5,83.25 67.2,83.25 J9.7
08  (via drill 0.7)
  Top 0.305: R40.1 44.88,56 v45.62,56.75
  Top 0.406: J1.8 108.44,84 107,84 105.75,85.25 98,85.25 96.61,83.86 J3.8 95.72,84 95,84 93.5,85.5 87.62,85.5 86.38,84.26 J5.8 84.5,84.25 83.38,85.38 78.12,85.38 76.86,84.11 J7.8 75.6,84.5 75.25,84.5 74,85.75 68,85.75 66.71,84.46 J9.8 65.66,84.25 64.25,84.25 58.75,78.75 58.75,42 53.25,36.5 16.25,36.5 10,42.75 10,166 11,167 66.75,167 67.97,168.22 J11.8 73.53,168.22 74.5,167.25 77,167.25 78,168.25 78.35,168.25 J14.8 83.84,168.41 85.25,167 87.5,167 88.74,168.24 J16.8 93.64,168.24 95.25,166.62 97.25,166.62 98.12,167.5 99.04,167.5 J18.8 106.07,167.8 106.62,167.25 109.12,167.25 110.38,168.5 111.06,168.5 J20.8
  Bottom 0.305: RN1.16 43.55,54.67 v45.62,56.75 47.38,58.5 47.38,58.62 50.88,62.12 50.88,66.12 64.25,79.5 64.25,83.75 64.75,84.25 65.66,84.25 J9.8
09  (via drill 0.7)
  Top 0.305: R41.1 45,57.38 v45.88,58.25
  Top 0.406: J1.9 110.94,86.5 110.25,86.5 109,85.25 107,85.25 105.85,86.4 J3.9 98,86 97.75,86 97,85.25 95,85.25 93.45,86.8 J5.9 88.04,86.62 87.25,86.62 86.12,85.5 84.75,85.5 83.12,87.12 79.38,87.12 78.9,86.65 J7.9 77.38,85.5 75.25,85.5 73.75,87 J9.9 67.16,85.75 64.5,85.75 57.75,79 57.75,42.5 52.5,37.25 16.5,37.25 10.75,43 10.75,164.75 11.68,165.68 J11.9 66.43,165.68 67.62,166.88 73.62,166.88 74.62,165.88 J14.9 76.62,165.87 77.75,167 83.88,167 85.12,165.75 86.72,165.75 J16.9 87.2,165.7 88.38,166.88 93.62,166.88 95.12,165.38 96.69,165.38 J18.9 97.26,165.26 98.5,166.5 106,166.5 106.5,166 J20.9
  Bottom 0.305: RN2.9 43.67,58.95 44.38,58.25 v45.88,58.25 50,62.38 50,66.25 63.62,79.88 63.62,84.88 64.31,85.56 66.97,85.56 J9.9
10  (via drill 0.7)
  Top 0.305: R42.1 44.5,58.75 v45,59.25
  Top 0.406: J1.10 108.25,86.75 106.75,86.75 105.75,87.75 97.75,87.75 96.4,86.4 J3.10 95.75,86.5 95,86.5 93.5,88 87.5,88 86.3,86.8 J5.10 85.6,86.88 85,86.88 83.88,88 78.25,88 76.9,86.65 J7.10 75.39,87.25 75,87.25 74,88.25 68,88.25 66.75,87 J9.10 65.62,86.75 64.5,86.75 56.75,79 56.75,42.75 52,38 17,38 11.5,43.5 11.5,163.75 12.25,164.5 67,164.5 68.18,165.68 J11.10 73.7,165.68 74.75,164.62 76.75,164.62 77.62,165.5 78.14,165.5 J14.10 83.75,165.87 85.12,164.5 87.5,164.5 88.5,165.5 89.12,165.5 J16.10 93.43,165.7 95.12,164 97.5,164 98.5,165 99.08,165 J18.10 105.74,165.26 106.38,164.62 109.72,164.62 J20.10
  Bottom 0.305: RN2.10 43.88,59.75 44.38,59.25 v45,59.25 45.62,59.25 49,62.62 49,66.88 62.88,80.75 62.88,85.12 64.38,86.62 65.5,86.62 J9.10
11  (via drill 0.7)
  Top 0.305: R43.1 45.12,60.12 v45.55,60.55
  Top 0.406: J1.11 110.9,89 110.5,89 109.25,87.75 107,87.75 105.81,88.94 J3.11 98.21,88.75 97.5,88.75 96.5,87.75 95,87.75 93.41,89.34 J5.11 88.12,89.25 87.5,89.25 86.38,88.12 84.88,88.12 83.81,89.19 J7.11 77.34,88 75.5,88 73.96,89.54 J9.11 67.12,88.25 64.5,88.25 56,79.75 56,43.25 51.5,38.75 17.5,38.75 12.25,44 12.25,162 13.39,163.14 J11.11 66.51,163.14 67.62,164.25 73.75,164.25 74.75,163.25 75.89,163.25 J14.11 76.71,163.33 78,164.62 83.25,164.62 84.75,163.12 86.74,163.12 J16.11 87.41,163.16 88.62,164.38 93.38,164.38 95,162.75 96.77,162.75 J18.11
  Bottom 0.305: RN2.11 v45.55,60.55 48.25,63.25 48.25,67.5 62.12,81.38 62.12,85.88 64.5,88.25 67.12,88.25 J9.11
12  (via drill 0.7)
  Top 0.305: R44.1 44.88,61.5 v45.12,61.75
  Top 0.406: J1.12 108.29,89.25 106.75,89.25 105.75,90.25 97.75,90.25 96.44,88.94 J3.12 95.8,89 94.75,89 93.25,90.5 87,90.5 85.84,89.34 J5.12 85.64,89.38 84.88,89.38 83.75,90.5 78.25,90.5 76.94,89.19 J7.12 75.93,89.25 75.25,89.25 73.75,90.75 68,90.75 66.79,89.54 J9.12 65.83,89.5 64.25,89.5 55.25,80.5 55.25,43.75 51,39.5 18.5,39.5 13,45 13,161 13.75,161.75 66.5,161.75 67.89,163.14 J11.12 73.61,163.14 74.75,162 77.18,162 J14.12 83.04,163.33 84.5,161.88 87.38,161.88 88.62,163.12 89.28,163.12 J16.12 93.34,163.16 95.12,161.38 97.5,161.38 98.5,162.38 99,162.38 J18.12
  Bottom 0.305: RN2.12 44.73,61.35 v45.12,61.75 47.62,64.25 47.62,67.88 61.5,81.75 61.5,86.5 64.5,89.5 65.83,89.5 J9.12
13  (via drill 0.7)
  Top 0.305: R45.1 45,62.88 46.69,64.56 46.69,66.56 v46.75,66.62
  Top 0.406: J1.13 109.61,90.25 107,90.25 105.77,91.48 J3.13 98.17,91.25 97.5,91.25 96.5,90.25 95.25,90.25 93.62,91.88 J5.13 88.08,91.75 87.25,91.75 86.25,90.75 85,90.75 84.02,91.73 J7.13 77.3,90.5 75.25,90.5 73.67,92.08 J9.13 67.08,90.75 64.25,90.75 54.5,81 54.5,44 50.75,40.25 18.75,40.25 13.75,45.25 13.75,159.75 14.6,160.6 J11.13 66.47,160.6 67.62,161.75 73.75,161.75 74.75,160.75 75.93,160.75 J14.13 76.92,160.79 78.12,162 83,162 84.38,160.62 86.77,160.62 J16.13 87.49,160.62 88.75,161.88 92.88,161.88 94.62,160.12 96.75,160.12 J18.13
  Bottom 0.305: RN2.13 44.27,62.15 46.75,64.62 v46.75,66.62 46.75,67.88 60.75,81.88 60.75,87.25 64.19,90.69 67.02,90.69 J9.13
14  (via drill 0.7)
  Top 0.305: R46.1 44.75,64.25 v45.5,65
  Top 0.406: J1.14 108.33,91.75 106.75,91.75 105.75,92.75 98,92.75 96.73,91.48 J3.14 95.59,91.75 95,91.75 93.5,93.25 87.25,93.25 85.88,91.88 J5.14 85.55,92 85,92 84,93 78,93 76.73,91.73 J7.14 75.97,91.75 75.25,91.75 73.75,93.25 68,93.25 66.83,92.08 J9.14 65.54,91.75 64,91.75 53.75,81.5 53.75,44.25 50.5,41 19,41 14.5,45.5 14.5,158.25 15.5,159.25 66.75,159.25 68.1,160.6 J11.14 73.9,160.6 74.62,159.88 75.25,159.88 75.5,159.62 76.88,159.62 78.04,160.79 J14.14 82.62,160.79 84.04,159.38 87.88,159.38 88.88,160.38 89.07,160.38 J16.14 91.76,160.62 93.62,158.75 97.91,158.75 J18.14
  Bottom 0.305: RN2.14 43.58,62.95 44,63.38 44.38,63.38 44.75,63.75 44.88,63.75 45.5,64.38 v45.5,65 45.5,67.5 60.12,82.12 60.12,87.88 64,91.75 65.54,91.75 J9.14
15  (via drill 0.7)
  Top 0.305: R47.1 43.5,65.62 v44.5,66.62
  Top 0.406: J1.15 109.82,93 106.75,93 105.73,94.02 J3.15 98.13,93.75 97.75,93.75 96.75,92.75 95.25,92.75 93.58,94.42 J5.15 88.04,94.25 87.25,94.25 86.25,93.25 85,93.25 83.98,94.27 J7.15 78.02,94.27 76.75,93 75.25,93 73.63,94.62 J9.15 67.04,93.25 64.25,93.25 53,82 53,44.5 50.25,41.75 19.5,41.75 15.25,46 15.25,156.75 16.56,158.06 J11.15 66.56,158.06 67.75,159.25 74.97,159.25 J14.15 76.88,158.25 78,159.38 82.88,159.38 84.12,158.12 86.73,158.12 J16.15
  Bottom 0.305: RN2.15 43.62,63.75 44.5,64.62 v44.5,66.62 44.5,67.38 59.38,82.25 59.38,88.38 64.12,93.12 66.92,93.12 J9.15
16  (via drill 0.7)
  Top 0.305: R48.1 43.15,67.28 v44.31,68.44
  Top 0.406: J1.16 108.37,94.25 106.75,94.25 105.75,95.25 97.5,95.25 96.27,94.02 J3.16 95.62,94.25 94.75,94.25 93.25,95.75 87.25,95.75 85.92,94.42 J5.16 85.59,94.5 85,94.5 84,95.5 78,95.5 76.77,94.27 J7.16 75.76,94.5 74.75,94.5 73.5,95.75 68,95.75 66.87,94.62 J9.16 65.75,94.5 64.5,94.5 52.25,82.25 52.25,45 49.75,42.5 20,42.5 16,46.5 16,155.75 17,156.75 66.75,156.75 68.06,158.06 J11.16 74.32,158.06 75.38,157 76.62,157 77.88,158.25 J14.16 82.87,158.25 84.25,156.88 88.11,156.88 J16.16
  Bottom 0.305: RN2.16 43.2,67.33 v44.31,68.44 46.5,70.62 47,70.62 58.62,82.25 58.62,88.62 64.5,94.5 65.75,94.5 J9.16
17  (via drill 0.7)
  Top 0.305: R49.1 46,71 v49,74
  Top 0.406: J1.17 110.78,96.5 110.25,96.5 109.25,95.5 106.75,95.5 105.69,96.56 J3.17 98.09,96.25 97.25,96.25 96.25,95.25 95,95.25 93.29,96.96 J5.17 87.75,96.5 87,96.5 86.25,95.75 84.75,95.75 83.69,96.81 J7.17 77.81,96.81 76.5,95.5 74.75,95.5 73.09,97.16 J9.17 67.25,96 64.75,96 51.5,82.75 51.5,45.25 49.5,43.25 20.25,43.25 16.75,46.75 16.75,155 17.27,155.52 J11.17 66.52,155.52 67.62,156.62 74.25,156.62 75.12,155.75 75.93,155.75 J14.17
  Bottom 0.305: RN3.9 45.17,75.33 46,74.5 49,74.5 | 49,74.5 57.75,83.25 57.75,89 64.75,96 67.25,96 J9.17 | v49,74 49,74.5
18  (via drill 0.7)
  Top 0.305: R50.1 45.62,72.38 v48.75,75.5
  Top 0.406: J1.18 108.41,96.75 106.75,96.75 105.75,97.75 97.75,97.75 96.56,96.56 J3.18 95.8,96.5 95.25,96.5 93.5,98.25 87.25,98.25 85.96,96.96 J5.18 84.63,98 78,98 76.81,96.81 J7.18 75.93,96.75 75.25,96.75 73.5,98.5 68,98.5 66.66,97.16 J9.18 65.71,97 64.5,97 50.75,83.25 50.75,45.5 49.25,44 20.75,44 17.5,47.25 17.5,153.5 18.25,154.25 66.75,154.25 68.02,155.52 J11.18 73.73,155.52 74.75,154.5 76.62,154.5 77.62,155.5 78.3,155.5 J14.18
  Bottom 0.305: RN3.10 45.38,76.12 46,75.5 v48.75,75.5 56.75,83.5 56.75,89.25 64.5,97 65.71,97 J9.18
19
  Top 0.305: 50,77.25 49.75,77 49.25,77 48.75,76.5 48.25,76.5 45.5,73.75 R51.1
  Top 0.406: J1.19 110.74,99 110,99 109,98 107,98 105.9,99.1 J3.19 97.8,98.5 97.5,98.5 96.75,97.75 95.25,97.75 93.5,99.5 J5.19 87.5,99.5 86.25,98.25 85.25,98.25 84.15,99.35 J7.19 77.85,99.35 76.5,98 75.25,98 73.55,99.7 J9.19 67.21,98.5 64.75,98.5 50,83.75 50,77.25 50,46 48.75,44.75 21,44.75 18.25,47.5 18.25,152 19.5,153.25 64.25,153.25 64.52,152.98 J11.19 66.48,152.98 67.75,154.25 73.62,154.25 74.62,153.25 75.89,153.25 J14.19
  Bottom 0.305: RN3.11 45.58,76.92 46,76.5 48.75,76.5 56,83.75 56,89.75 64.75,98.5 67.21,98.5 J9.19
20  (via drill 0.7)
  Top 0.305: R52.1 45.88,75.12 v48.12,77.38
  Top 0.406: J1.20 107,99.25 106,100.25 97.75,100.25 96.6,99.1 J3.20 95.7,99.25 95.25,99.25 93.75,100.75 87,100.75 85.75,99.5 J5.20 85.42,99.75 85.25,99.75 84.5,100.5 78,100.5 76.85,99.35 J7.20 75.84,99.5 75.25,99.5 73.75,101 68,101 66.7,99.7 J9.20 65.67,99.5 58.25,99.5 55.5,102.25 55.5,149.25 58,151.75 66.75,151.75 67.98,152.98 J11.20 73.9,152.98 74.88,152 77.34,152 J14.20
  Bottom 0.305: RN3.12 45.52,77.72 46.25,77 47.75,77 v48.12,77.38 48.5,77.75 55.25,84.5 55.25,90 64.75,99.5 65.67,99.5 J9.20
21  (via drill 0.7)
  Top 0.305: R53.1 45.5,76.5 v47,78
  Top 0.406: J11.21 57.69,150.44 56.25,149 56.25,102.75 58,101 67.17,101 J9.21 73.76,102.24 75.5,100.5 76.75,100.5 78.14,101.89 J7.21 84.11,101.89 85.25,100.75 86,100.75 87,101.75 87.92,101.75 J5.21 93.71,102.04 95.25,100.5 96.5,100.5 97.25,101.25 98.01,101.25 J3.21 106.11,101.64 107.25,100.5 109,100.5 110.25,101.75 110.95,101.75 J1.21
  Bottom 0.305: RN3.13 45.73,78.53 46.25,78 v47,78 54.25,85.25 54.25,90.5 64.75,101 67.17,101 J9.21
22  (via drill 0.7)
  Top 0.305: R54.1 45.5,78 v46.83,79.33
  Top 0.406: J11.22 67.94,150.44 66.75,149.25 58.5,149.25 57,147.75 57,103.75 58.5,102.25 J9.22 | J9.22 | J9.22 66.75,102.25 68,103.5 74.38,103.5 J7.22 76.89,101.89 78.25,103.25 83.75,103.25 85,102 85.63,102 J5.22 85.79,102.04 87,103.25 93.75,103.25 95.25,101.75 95.75,101.75 J3.22 96.64,101.64 97.75,102.75 106.25,102.75 107,102 108.24,102 J1.22
  Bottom 0.305: RN3.14 45.75,79.33 v46.83,79.33 53.5,86 53.5,91.25 64.5,102.25 J9.22
23  (via drill 0.7)
  Top 0.305: R55.1 45.5,79.5 v47.25,81.25
  Top 0.406: J11.23 58.4,147.9 57.75,147.25 57.75,104.5 58.75,103.5 67.13,103.5 J9.23 73.22,104.78 73.25,104.75 74,104.75 75.5,103.25 77.35,103.25 J7.23 84.07,104.43 85.25,103.25 86,103.25 87.25,104.5 88.13,104.5 J5.23 93.67,104.58 95.25,103 97,103 97.5,103.5 97.72,103.5 J3.23 106.32,104.18 107.5,103 109.25,103 110.25,104 110.66,104 J1.23
  Bottom 0.305: RN3.15 46.12,80.12 v47.25,81.25 52.5,86.5 52.5,91.5 64.5,103.5 67.13,103.5 J9.23
24  (via drill 0.7)
  Top 0.305: R56.1 45.5,81 v45.88,81.38
  Top 0.406: J11.24 67.9,147.9 66.5,146.5 59.75,146.5 58.5,145.25 58.5,106 59.75,104.75 65.84,104.75 J9.24 66.78,104.78 68,106 73.75,106 75,104.75 75.67,104.75 J7.24 | 75.92,104.5 J7.24 | J1.24 108.37,104.25 107.5,104.25 106.25,105.5 97.75,105.5 96.43,104.18 J3.24 95.53,104.5 95,104.5 93.75,105.75 87,105.75 85.83,104.58 J5.24 85.5,104.75 85,104.75 84,105.75 78.25,105.75 76.93,104.43 J7.24
  Bottom 0.305: RN3.16 45.42,80.92 v45.88,81.38 51.75,87.25 51.75,91.75 64.75,104.75 65.84,104.75 J9.24
25  (via drill 0.7)
  Top 0.305: R57.1 45.75,82.75 v48.5,85.5
  Top 0.406: J11.25 60.36,145.36 59.25,144.25 59.25,107.25 60.5,106 67.09,106 J9.25 73.43,107.32 75,105.75 77.31,105.75 J7.25 84.03,106.97 85,106 86.25,106 87.25,107 88.09,107 J5.25 93.63,107.12 95.25,105.5 96.5,105.5 97.25,106.25 97.93,106.25 J3.25 106.28,106.72 107.5,105.5 108.75,105.5 110,106.75 110.87,106.75 J1.25
  Bottom 0.305: RN4.9 46.3,85.7 46.5,85.5 48,85.5 v48.5,85.5 51,88 51,92.5 64.5,106 67.09,106 J9.25
26  (via drill 0.7)
  Top 0.305: R58.1 45.75,84.25 v48.62,87.12
  Top 0.406: J11.26 68.19,145.19 67,144 62.25,144 60,141.75 60,108.5 61.25,107.25 65.8,107.25 J9.26 65.87,107.37 67,108.5 73.25,108.5 74.75,107 75.96,107 J7.26 76.47,106.97 77.75,108.25 84,108.25 85,107.25 85.54,107.25 J5.26 85.87,107.12 87,108.25 93.75,108.25 95.25,106.75 95.83,106.75 J3.26 96.22,106.72 97.5,108 106.5,108 107.5,107 108.32,107 J1.26
  Bottom 0.305: RN4.10 46.25,86.5 46.5,86.25 47.75,86.25 v48.62,87.12 49.75,88.25 50.25,88.75 50.25,92.75 64.75,107.25 65.8,107.25 J9.26
27  (via drill 0.7)
  Top 0.305: R59.1 45.7,85.75 v47.25,87.3
  Top 0.406: J9.27 73.39,109.86 75,108.25 76.75,108.25 78,109.5 J7.27 83.74,109.51 84.75,108.5 86.25,108.5 87.25,109.5 88.05,109.5 J5.27 93.59,109.66 95.25,108 96.5,108 97.5,109 98.14,109 J3.27 106.49,109.26 107.5,108.25 109.25,108.25 110,109 110.58,109 J1.27
  Bottom 0.305: RN4.11 v47.25,87.3 47.3,87.3 48,88 49.5,89.5 49.5,93.25 64.75,108.5 67.05,108.5 J9.27
28  (via drill 0.7)
  Top 0.305: R60.1 45.5,87.25 v47.38,89.12
  Top 0.406: J9.28 66.61,109.86 67.75,111 73.5,111 75,109.5 J7.28 76.51,109.51 77.75,110.75 83.75,110.75 84.75,109.75 85.58,109.75 J5.28 85.67,109.67 86.17,109.67 87.5,111 93.5,111 95,109.5 95.62,109.5 J3.28 96.01,109.26 97.25,110.5 106.5,110.5 107.5,109.5 108.36,109.5 J1.28
  Bottom 0.305: RN4.12 45.4,88.1 45.5,88 46.25,88 v47.38,89.12 48.75,90.5 48.75,93.5 65,109.75 65.76,109.75 J9.28
29  (via drill 0.7)
  Top 0.305: R61.1 45.75,88.75 v45.9,88.9
  Top 0.406: J9.29 73.6,112.4 75.25,110.75 76.75,110.75 78.05,112.05 J7.29 83.95,112.05 85,111 86.25,111 87.25,112 88.01,112 J5.29 93.55,112.2 95.25,110.5 96.25,110.5 97.25,111.5 98.1,111.5 J3.29 106.2,111.8 107.25,110.75 109.79,110.75 J1.29
  Bottom 0.305: RN4.13 v45.9,88.9 47.75,90.75 47.75,94 64.75,111 67.01,111 J9.29
30  (via drill 0.7)
  Top 0.305: R62.1 46,90.25 v46.75,91
  Top 0.406: J9.30 66.15,112.4 67.5,113.75 73.5,113.75 75,112.25 75.79,112.25 J7.30 76.8,112.05 78.25,113.5 83.75,113.5 85,112.25 85.62,112.25 J5.30 86.45,112.2 87.75,113.5 93.75,113.5 95.25,112 95.66,112 J3.30 96.3,111.8 97.5,113 106.5,113 107.5,112 108.4,112 J1.30
  Bottom 0.305: J9.30 64.4,112.4 46.75,94.75 v46.75,91 45.5,89.75 44.38,89.75 RN4.14
31  (via drill 0.7)
  Top 0.305: R63.1 44.52,91.78 v45.75,93
  Top 0.406: J9.31 73.56,114.94 75.25,113.25 76.5,113.25 77.84,114.59 J7.31 83.91,114.59 85,113.5 86.25,113.5 87.5,114.75 J5.31 93.76,114.74 95.5,113 96.5,113 97.5,114 98.06,114 J3.31 106.66,114.34 107.75,113.25 109.5,113.25 110.5,114.25 110.75,114.25 J1.31
  Bottom 0.305: RN4.15 45,90.5 45.75,91.25 v45.75,93 45.75,95.5 64,113.75 67.22,113.75 J9.31
32  (via drill 0.7)
  Top 0.305: R64.1 44.52,94.8 v44.33,95
  Top 0.406: J9.32 66.44,114.94 67.75,116.25 73.75,116.25 75.25,114.75 75.83,114.75 J7.32 76.84,114.59 78,115.75 84,115.75 85,114.75 J5.32 85.99,114.74 87.25,116 93.75,116 95.41,114.34 J3.32 96.34,114.34 97.5,115.5 106.5,115.5 107.5,114.5 J1.32
  Bottom 0.305: RN4.16 v44.33,95 44.33,95.33 44.75,95.75 64,115 65.81,115 J9.32
33  (via drill 0.7)
  Top 0.305: R65.1 50.25,103 52.62,105.38 v52.62,105.5
  Top 0.406: J9.33 73.77,117.48 75.25,116 77.4,116 J7.33 83.87,117.13 85,116 86.25,116 87.25,117 87.93,117 J5.33 93.72,117.28 95.5,115.5 96.25,115.5 97.25,116.5 98.02,116.5 J3.33 106.37,116.88 107.5,115.75 109.25,115.75 110.25,116.75 110.71,116.75 J1.33
  Bottom 0.305: RN5.9 47.67,106.95 48.62,106 52.62,106 | 52.62,106 53,106 63.12,116.12 67.06,116.12 J9.33 | v52.62,105.5 52.62,106
34  (via drill 0.7)
  Top 0.305: R66.1 50,104.5 v52.62,107.12
  Top 0.406: J9.34 65.87,117.62 67,118.75 73.5,118.75 75,117.25 75.87,117.25 J7.34 76.13,117.13 77.5,118.5 83.5,118.5 84.75,117.25 85.64,117.25 J5.34 86.03,117.28 87.25,118.5 93.5,118.5 95,117 95.73,117 J3.34 96.38,116.88 97.5,118 106.5,118 107.5,117 108.42,117 J1.34
  Bottom 0.305: RN5.10 47.88,107.75 48.5,107.12 v52.62,107.12 53.12,107.12 53.19,107.19 63.5,117.5 65.85,117.5 J9.34
35  (via drill 0.7)
  Top 0.305: R67.1 49.62,106 v51.75,108.12
  Top 0.406: J1.35 110.92,119.5 110,119.5 108.75,118.25 107.75,118.25 106.58,119.42 J3.35 97.98,119 97.25,119 96.5,118.25 95,118.25 93.43,119.82 J5.35 88.14,119.75 87.5,119.75 86.25,118.5 85,118.5 83.83,119.67 J7.35
  Bottom 0.305: RN5.11 48.2,108.55 48.62,108.12 50.62,108.12 v51.75,108.12 52.62,108.12 63.25,118.75 74.88,118.75 75.25,118.38 77.24,118.38 J7.35
36  (via drill 0.7)
  Top 0.305: R68.1 49,107.5 v50.62,109.12
  Top 0.406: J1.36 108.27,119.75 107.5,119.75 106.5,120.75 98,120.75 96.67,119.42 J3.36 95.53,119.75 94.75,119.75 93.5,121 87.5,121 86.32,119.82 J5.36 85.49,120 85,120 84,121 77,121 75.99,119.99 J7.36
  Bottom 0.305: RN5.12 48.52,109.35 48.75,109.12 v50.62,109.12 51.75,109.12 62.25,119.62 75.95,119.62 J7.36
37  (via drill 0.7)
  Top 0.305: R69.1 48.75,109.25 v49.5,110
  Top 0.406: J1.37 110.88,122 110.5,122 109.25,120.75 108,120.75 106.79,121.96 J3.37 98.19,121.75 97.75,121.75 96.75,120.75 95,120.75 93.39,122.36 J5.37 87.85,122 87.25,122 86.25,121 85.25,121 84.04,122.21 J7.37
  Bottom 0.305: RN5.13 47.98,110.15 48.12,110 v49.5,110 50.88,110 61.88,121 77.32,121 J7.37
38  (via drill 0.7)
  Top 0.305: R70.1 47.92,110.75 v48.38,110.95
  Top 0.406: J1.38 108.31,122.25 107.5,122.25 106.5,123.25 97.5,123.25 96.21,121.96 J3.38 95.56,122.25 94.5,122.25 93,123.75 88,123.75 86.61,122.36 J5.38 85.53,122.5 85.25,122.5 84.25,123.5 77.5,123.5 76.21,122.21 J7.38
  Bottom 0.305: RN5.14 v48.38,110.95 | v48.38,110.95 48.42,110.95 48.5,110.88 48.62,110.88 | 48.62,110.88 50.25,110.88 61.62,122.25 75.95,122.25 J7.38 | v48.38,110.95 48.55,110.95 48.62,110.88
39  (via drill 0.7)
  Top 0.305: R71.1 48.88,112.5 v49.62,111.75
  Top 0.406: J1.39 110.84,124.5 110.25,124.5 109.25,123.5 107.5,123.5 106.5,124.5 J3.39 98.15,124.25 97.25,124.25 96.25,123.25 95,123.25 93.35,124.9 J5.39 88.06,124.75 87.25,124.75 86.25,123.75 85,123.75 84,124.75 J7.39
  Bottom 0.305: J7.39 77.41,123.62 61.88,123.62 50,111.75 v49.62,111.75 49.5,111.88 47.75,111.88 47.62,111.75 RN5.15
40  (via drill 0.7)
  Top 0.305: R72.1 50.5,113.75 v50.56,113.69
  Top 0.406: J1.40 108.35,124.75 107.25,124.75 106.25,125.75 97.5,125.75 96.25,124.5 J3.40 95.6,124.75 94.75,124.75 93.25,126.25 87.25,126.25 85.9,124.9 J5.40 84.32,126.25 77.5,126.25 J7.40
  Bottom 0.305: J7.40 61.62,124.75 v50.56,113.69 49.88,113 47.88,113 47.42,112.55 RN5.16
41  (via drill 0.7)
  Top 0.305: R73.1 49.12,116 v50.12,117
  Top 0.406: J5.41 93.31,127.44 95,125.75 96.25,125.75 97.25,126.75 98.11,126.75 J3.41 106.46,127.04 107.5,126 109,126 110,127 110.8,127 J1.41
  Bottom 0.305: RN6.9 47.8,117.58 48.38,117 v50.12,117 52.75,117 62,126.25 87.02,126.25 J5.41
42  (via drill 0.7)
  Top 0.305: R74.1 48.25,117.25 v48.88,117.88
  Top 0.406: J5.42 85.69,127.44 87,128.75 93.25,128.75 94.75,127.25 95.65,127.25 J3.42 96.29,127.04 97.5,128.25 106.25,128.25 107.25,127.25 108.39,127.25 J1.42
  Bottom 0.305: RN6.10 48.38,118.38 v48.88,117.88 52,117.88 61.5,127.38 85.61,127.38 J5.42
43  (via drill 0.7)
  Top 0.305: R75.1 v50.38,118.75
  Top 0.406: J5.43 93.27,129.98 95,128.25 96.25,128.25 97.25,129.25 98.07,129.25 J3.43 106.67,129.58 107.75,128.5 109,128.5 110,129.5 110.76,129.5 J1.43
  Bottom 0.305: RN6.11 48.33,119.17 48.75,118.75 v50.38,118.75 51.38,118.75 61.38,128.75 86.98,128.75 J5.43
44  (via drill 0.7)
  Top 0.305: R76.1 48.75,120 v49,119.75
  Top 0.406: J5.44 85.98,129.98 87.25,131.25 93.5,131.25 95.25,129.5 95.78,129.5 J3.44 96.33,129.58 97.5,130.75 106.75,130.75 107.75,129.75 108.43,129.75 J1.44
  Bottom 0.305: RN6.12 48.52,119.97 48.75,119.75 v49,119.75 51.5,119.75 61.75,130 85.65,130 J5.44
45  (via drill 0.7)
  Top 0.305: R77.1 48,121.25 48.62,120.62 50.12,120.62 v50.25,120.75
  Top 0.406: J5.45 93.48,132.52 95,131 96.5,131 97.25,131.75 98.03,131.75 J3.45 106.63,132.12 107.75,131 109.25,131 110.25,132 110.72,132 J1.45
  Bottom 0.305: RN6.13 47.98,120.78 48,120.75 48.5,120.75 48.62,120.62 49.75,120.62 49.88,120.5 50,120.5 v50.25,120.75 50.88,120.75 61.38,131.25 86.94,131.25 J5.45
46  (via drill 0.7)
  Top 0.305: R78.1 47.83,122.75 v49,121.58
  Top 0.406: J5.46 86.02,132.52 87.25,133.75 93.75,133.75 95.25,132.25 95.72,132.25 J3.46 96.37,132.12 97.5,133.25 107,133.25 107.75,132.5 108.22,132.5 J1.46
  Bottom 0.305: RN6.14 v49,121.58 49.95,121.58 52.88,124.5 52.88,124.62 57,128.75 57.12,128.75 61.12,132.75 85.44,132.75 J5.46
47  (via drill 0.7)
  Top 0.305: R79.1 51.38,124.25 v51.81,124.69
  Top 0.406: J5.47 93.69,135.06 95.25,133.5 96.5,133.5 97.5,134.5 98.24,134.5 J3.47 106.84,134.66 108,133.5 109,133.5 110.25,134.75 110.93,134.75 J1.47
  Bottom 0.305: RN6.15 48.12,122.38 48.25,122.5 49.62,122.5 v51.81,124.69 61,133.88 87.03,133.88 J5.47
48  (via drill 0.7)
  Top 0.305: R80.1 51.5,125.75 v51.88,126.12
  Top 0.406: J5.48 86.56,135.06 87.75,136.25 93.75,136.25 95.25,134.75 95.77,134.75 J3.48 96.41,134.66 97.75,136 106.5,136 107.75,134.75 108.39,134.75 J1.48
  Bottom 0.305: RN6.16 48.92,123.17 v51.88,126.12 | 56,130.25 56,130.38 60.88,135.25 85.48,135.25 J5.48
  Bottom 0.406: 56,130.25 v51.88,126.12
49  (via drill 0.7)
  Top 0.305: R81.1 51.75,128.5 v54.5,131.25
  Top 0.406: J5.49 93.65,137.6 95.25,136 96.5,136 97.75,137.25 98.34,137.25 J3.49 106.55,137.2 107.75,136 109,136 110,137 110.25,137 110.5,137.25 110.89,137.25 J1.49
  Bottom 0.305: RN7.9 49.55,131.95 50.25,131.25 v54.5,131.25 54.5,131.5 59.38,136.38 86.99,136.38 J5.49
50  (via drill 0.7)
  Top 0.305: R82.1 51,130 v53.25,132.25
  Top 0.406: J1.50 108.3,137.5 107.5,137.5 106.5,138.5 97,138.5 95.86,137.36 J3.50 94.31,138.75 87.5,138.75 86.35,137.6 J5.50
  Bottom 0.305: RN7.10 49.75,132.75 50.25,132.25 v53.25,132.25 53.25,132.5 58.5,137.75 85,137.75 85.52,137.75 J5.50
51  (via drill 0.7)
  Top 0.305: R83.1 50.25,131.5 v52,133.25
  Top 0.406: J3.51 106.51,139.74 107.75,138.5 108.75,138.5 110,139.75 110.85,139.75 J1.51
  Bottom 0.305: RN7.11 49.95,133.55 50.25,133.25 v52,133.25 52.12,133.25 57.5,138.62 84,138.62 84.62,139.25 94.25,139.25 95,138.5 97.16,138.5 J3.51
52  (via drill 0.7)
  Top 0.305: R84.1 49.5,133 v50.75,134.25
  Top 0.406: J3.52 95.99,139.74 97.25,141 106.5,141 107.5,140 108.34,140 J1.52
  Bottom 0.305: RN7.12 48.9,134.35 49,134.25 v50.75,134.25 51.62,134.25 56.62,139.25 83.12,139.25 84,140.12 95.47,140.12 J3.52 95.84,139.75
53  (via drill 0.7)
  Top 0.305: R85.1 48.85,134.5 v49.5,135.15
  Top 0.406: J3.53 106.47,142.28 107.5,141.25 109,141.25 110,142.25 110.81,142.25 J1.53
  Bottom 0.305: RN7.13 v49.5,135.15 51.65,135.15 56.25,139.75 82.5,139.75 83.62,140.88 97,140.88 97.37,141.25 J3.53
54  (via drill 0.7)
  Top 0.305: R86.1 48.5,136 49.25,136.75 v51,136.75
  Top 0.406: J3.54 96.28,142.28 97.5,143.5 106.25,143.5 107.25,142.5 108.38,142.5 J1.54
  Bottom 0.305: RN7.14 48.45,135.95 49.25,136.75 v51,136.75 54.5,140.25 82.12,140.25 84.12,142.25 95.83,142.25 J3.54
55  (via drill 0.7)
  Top 0.305: R87.1 50,137.5 v50.25,137.75
  Top 0.406: J3.55 106.43,144.82 107.5,143.75 109,143.75 110.25,145 110.96,145 J1.55
  Bottom 0.305: J3.55 97.08,143.5 85.25,143.5 85.12,143.38 84.38,143.38 81.75,140.75 52.75,140.75 50.25,138.25 v50.25,137.75 49,137.75 48,136.75 RN7.15
56  (via drill 0.7)
  Top 0.305: R88.1 49,139 v49.25,138.75
  Top 0.406: J3.56 96.07,144.82 97.25,146 106.5,146 107.5,145 108.42,145 J1.56
  Bottom 0.305: J3.56 95.67,145 85.25,145 81.62,141.38 52.5,141.38 49.88,138.75 v49.25,138.75 48.5,138.75 47.3,137.55 RN7.16
57  (via drill 0.7)
  Top 0.305: R89.1 49.75,141.5 v50.75,142.75
  Top 0.406: J3.57 106.64,147.36 107.75,146.25 109,146.25 110.25,147.5 110.98,147.5 J1.57
  Bottom 0.305: RN8.9 47.55,143.95 48.75,142.75 v50.75,142.75 63.25,142.75 64,142 81,142 85.25,146.25 97.29,146.25 J3.57
58  (via drill 0.7)
  Top 0.305: R90.1 49,143 v49.75,143.75
  Top 0.406: J3.58 97,148.5 106.75,148.5 107.75,147.5 108.44,147.5 J1.58
  Bottom 0.305: RN8.10 47.5,144.75 48.5,143.75 v49.75,143.75 63.25,143.75 64.25,142.75 80.5,142.75 85.25,147.5 95.72,147.5 J3.58
59  (via drill 0.7)
  Top 0.305: R91.1 48.5,144.5 v48.75,144.75
  Top 0.406: J3.59 106.6,149.9 107.75,148.75 109.69,148.75 J1.59
  Bottom 0.305: RN8.11 47.95,145.55 v48.75,144.75 63,144.75 64.5,143.25 79.75,143.25 85.25,148.75 97.25,148.75 J3.59
60  (via drill 0.7)
  Top 0.305: R92.1 50,146 v50.25,145.75
  Top 0.406: J3.60 95.86,150.11 97,151.25 106.5,151.25 107.75,150 108.4,150 J1.60
  Bottom 0.305: RN8.12 47.9,146.35 48.5,145.75 v50.25,145.75 62.75,145.75 64.75,143.75 79,143.75 85.25,150 95.75,150 J3.60
61  (via drill 0.7)
  Top 0.305: R93.1 47.65,147.5 48,147.15 48.1,147.15 48.25,147 v50.75,147
  Bottom 0.305: J1.61 109.9,151.5 85.25,151.5 78,144.25 65,144.25 62.25,147 v50.75,147 48.25,147 48.1,147.15 RN8.13
62  (via drill 0.7)
  Top 0.305: R94.1 47.7,149 48.75,147.95 v49.75,147.95
  Bottom 0.305: RN8.14 v49.75,147.95 62.8,147.95 64.25,146.5 78.75,146.5 85.25,153 108.04,153 J1.62
63  (via drill 0.7)
  Top 0.305: R95.1 47.5,150.5 v48.75,149.25
  Bottom 0.305: RN8.15 48.25,148.75 v48.75,149.25 79.75,149.25 84.5,154 109.86,154 J1.63
64  (via drill 0.7)
  Top 0.305: R96.1 48.5,152 v48.75,151.75
  Bottom 0.305: RN8.16 46.83,150.57 48,151.75 v48.75,151.75 81.25,151.75 84.75,155.25 108.33,155.25 J1.64
+3V3
  Top 0.5: DIS1.J1.6 JP1.1
  Top 0.61: U13.4 218,35 221.38,31.62 221.38,24 214.5,17.12 214.5,17 206.75,17 203.5,13.75 203.5,11.55 DIS1.J1.6
  Bottom 0.5: JP1.1 203.46,4.29 C47.+
+5V  (via drill 0.7, 0.7 pad 0.25)
  Top 0.406: U8.18 U8.17 U8.16 U8.15 | C3.2 203.47,130.72 203.75,131 | 194.25,143.97 194.03,143.97 | C1.2 40.67,138.83 v41.25,138.25 | 199.45,46.25 201.95,46.25 R1.2 | C8.2 203.78,79.35 204,79.12
  Top 0.5: C5.2 20.52,49.88 v25.25,49.88 27.5,52 v30.5,52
